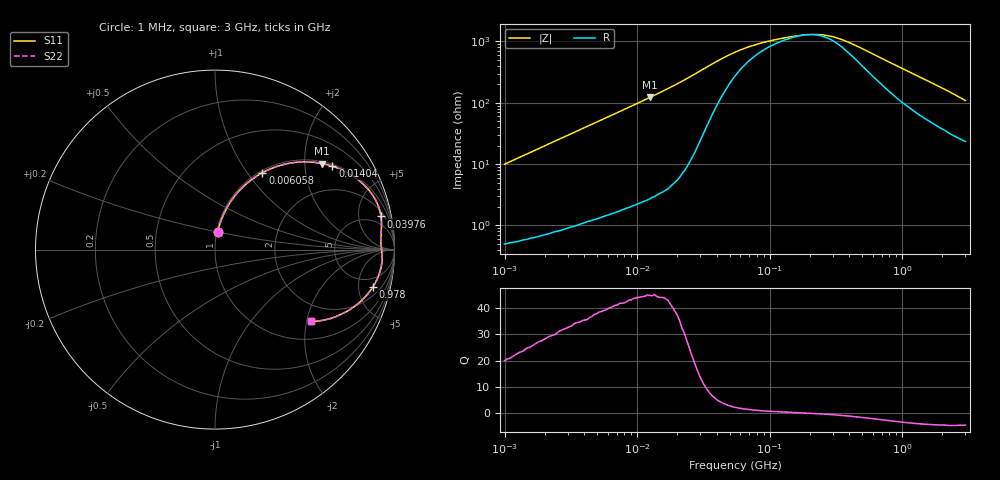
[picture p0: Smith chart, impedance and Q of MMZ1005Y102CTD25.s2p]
! S-Parameter Data Generated by TDK Corporation
! Copyright(C) 2025 TDK Corporation.
! All Rights Reserved.
! TDK P/N: MMZ1005Y102CTD25 (Chip Bead)
! Property: |Z|=1000ohm at 100MHz
! Size(LxWxT): 1x0.5x0.5mm
! Model Type: s2p (Touchstone File Format Version 1.0)
! Frequency: DC=Yes Start=1MHz Stop=3000MHz 202points Log-sweep
! Model Generated on Feb. 6, 2025
! Terms and conditions regarding TDK Simulation Models:
! 1)This simulation model is being provided solely for informational
!  purposes. Please refer to the specifications of the products in
!  terms of detailed characteristics of such products.
! 2)In no event shall TDK Corporation of any of its subsidiaries be
!  liable for any loss or damage arising, directly or indirectly,
!  from any information contained in this simulation model, including,
!  but not limited to loss or damages arising from any inaccuracies,
!  omissions or errors in connection with such information.
! 3)Any and all copyrights on this simulation model are owned by
!  TDK Corporation.  Duplication or redistribution of this simulation
!  model without prior written permission from TDK Corporation
!  is prohibited.
! 4)This simulation model is subject to any modification or change
!  without any prior notice.
! 5)Neither TDK Corporation nor any of its subsidiaries shall make any
!  warranty, express or implied, including but not limited to the
!  correctness, implied warranties of merchantability and fitness for
!  a particular purpose with respect to this simulation models.
! 6)The use of this simulation model shall be deemed to have consented
!  to the terms and conditions hereof.
! Port Assignments:
!  1 ---@@@--- 2
! Applicable Conditions:
!  Temperature = 25 degC
!  DC Bias Current = 0 A
!  Small Signal Operation
# Hz S MA R 50
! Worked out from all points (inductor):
!   201 points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, 1 MHz to 3 GHz, reference 50 ohm
!   read as one part in series: L = 1.58 uH near 1.041 MHz
!   highest Q = 44.8 at 12.45 MHz (marker M1), where L = 1.56 uH
!   self-resonance near 193.9 MHz
!   S11 on the Smith chart (normalised r, x): 1 MHz: 1.01, +0.20; 6.058 MHz: 1.03, +1.18; 14.04 MHz: 1.06, +2.77; 39.76 MHz: 2.78, +9.28; 978 MHz: 3.12, -7.11; 3 GHz: 1.47, -2.12
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1000000  0.09872 81.5  0.9902 -5.7  0.9902 -5.7  0.09872 81.5
2226959  0.2138 75.7  0.9696 -12.3  0.9696 -12.3  0.2138 75.7
3900413  0.3543 67.6  0.9251 -20.7  0.9251 -20.7  0.3543 67.6
6058321  0.5036 58.3  0.8514 -30.2  0.8514 -30.2  0.5036 58.3
8686058  0.6391 49.0  0.7544 -39.7  0.7544 -39.7  0.6391 49.0
1.245355e7  0.7654 38.8  0.6267 -49.9  0.6267 -49.9  0.7654 38.8
1.404268e7  0.802 35.4  0.5795 -53.3  0.5795 -53.3  0.802 35.4
1.461624e7  0.8133 34.3  0.5636 -54.4  0.5636 -54.4  0.8133 34.3
2.459509e7  0.9209 20.8  0.3551 -67.0  0.3551 -67.0  0.9209 20.8
3.976269e7  0.943 11.3  0.1997 -67.9  0.1997 -67.9  0.943 11.3
5.477226e7  0.9346 7.3  0.1398 -58.5  0.1398 -58.5  0.9346 7.3
7.852918e7  0.9275 4.4  0.1041 -43.7  0.1041 -43.7  0.9275 4.4
1.039275e8  0.9254 2.9  0.0888 -31.4  0.0888 -31.4  0.9254 2.9
1.49005e8  0.9261 1.2  0.07651 -14.5  0.07651 -14.5  0.9261 1.2
2.136344e8  0.9289 -0.5  0.0715 5.9  0.0715 5.9  0.9289 -0.5
2.716345e8  0.9314 -1.7  0.07444 21.9  0.07444 21.9  0.9314 -1.7
3.453811e8  0.9328 -3.2  0.08574 36.9  0.08574 36.9  0.9328 -3.2
8.005644e8  0.9162 -10.8  0.199 59.8  0.199 59.8  0.9162 -10.8
9.779672e8  0.9028 -13.5  0.2433 59.9  0.2433 59.9  0.9028 -13.5
1.782824e9  0.8226 -24.0  0.4164 53.4  0.4164 53.4  0.8226 -24.0
2.266846e9  0.7649 -29.5  0.5035 48.4  0.5035 48.4  0.7649 -29.5
3e9  0.6676 -36.9  0.6145 40.7  0.6145 40.7  0.6676 -36.9
